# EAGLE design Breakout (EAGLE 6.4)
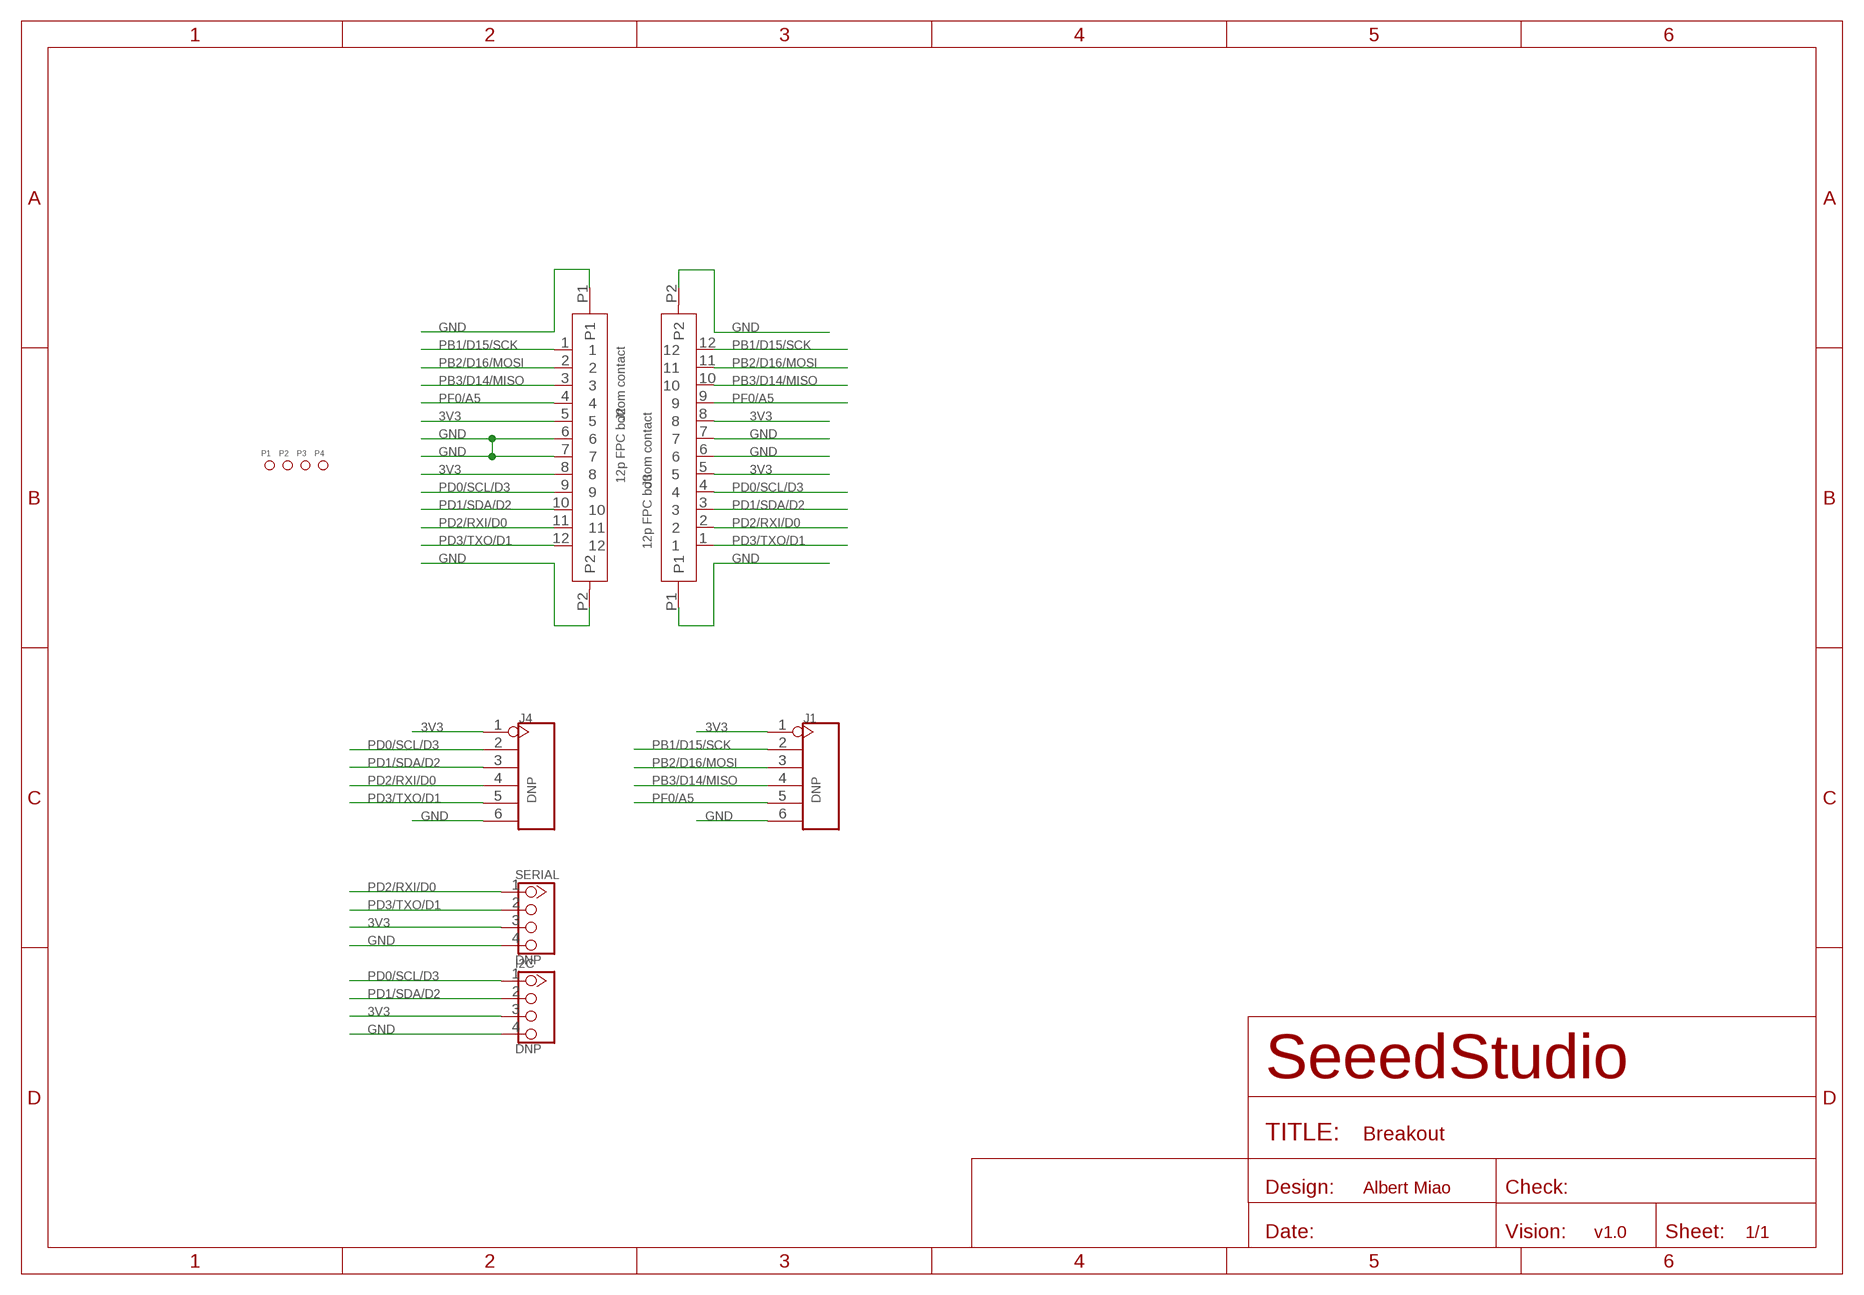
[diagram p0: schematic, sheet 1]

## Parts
I2C  DNP  TWIG-2.0-LEADED  [4P-LEADED-2.0]
J1  DNP  HEADER-6P-65/35MIL  [6P-2.54-65/35MIL]
J2  12p FPC bottom contact  FPC052002-12LT  [12P-0.5]
J3  12p FPC bottom contact  FPC052002-12LT  [12P-0.5]
J4  DNP  HEADER-6P-65/35MIL  [6P-2.54-65/35MIL]
P1  PAD-MARK  [ROUND-MARK-1.0]
P2  PAD-MARK  [ROUND-MARK-1.0]
P3  PAD-MARK  [ROUND-MARK-1.0]
P4  PAD-MARK  [ROUND-MARK-1.0]
SERIAL  DNP  TWIG-2.0-LEADED  [4P-LEADED-2.0]

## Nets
3V3: I2C.3 J1.1 J2.5 J2.8 J3.5 J3.8 J4.1 SERIAL.3
GND: I2C.4 J1.6 J2.6 J2.7 J2.P1 J2.P2 J3.6 J3.7 J3.P1 J3.P2 J4.6 SERIAL.4
PB1/D15/SCK: J1.2 J2.1 J3.12
PB2/D16/MOSI: J1.3 J2.2 J3.11
PB3/D14/MISO: J1.4 J2.3 J3.10
PD0/SCL/D3: I2C.1 J2.9 J3.4 J4.2
PD1/SDA/D2: I2C.2 J2.10 J3.3 J4.3
PD2/RXI/D0: J2.11 J3.2 J4.4 SERIAL.1
PD3/TXO/D1: J2.12 J3.1 J4.5 SERIAL.2
PF0/A5: J1.5 J2.4 J3.9

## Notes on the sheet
- Albert Miao
- v1.0

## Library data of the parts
I2C SERIAL = Connector:TWIG-2.0-LEADED
J1 J4 = Connector:HEADER-6P
J2 J3 = template:FPC052002-12LT
P1-P4 = Discrete:PAD-MARK; PARTNO: DNP

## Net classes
0 default: width 0.152 mm, drill 0.305 mm, clearance 0.152 mm
1 GND: width 0.152 mm, drill 0.305 mm, clearance 0.152 mm to class 0, clearance 0.152 mm
3 usbvcc: width 0.203 mm, drill 0.305 mm, clearance 0.203 mm

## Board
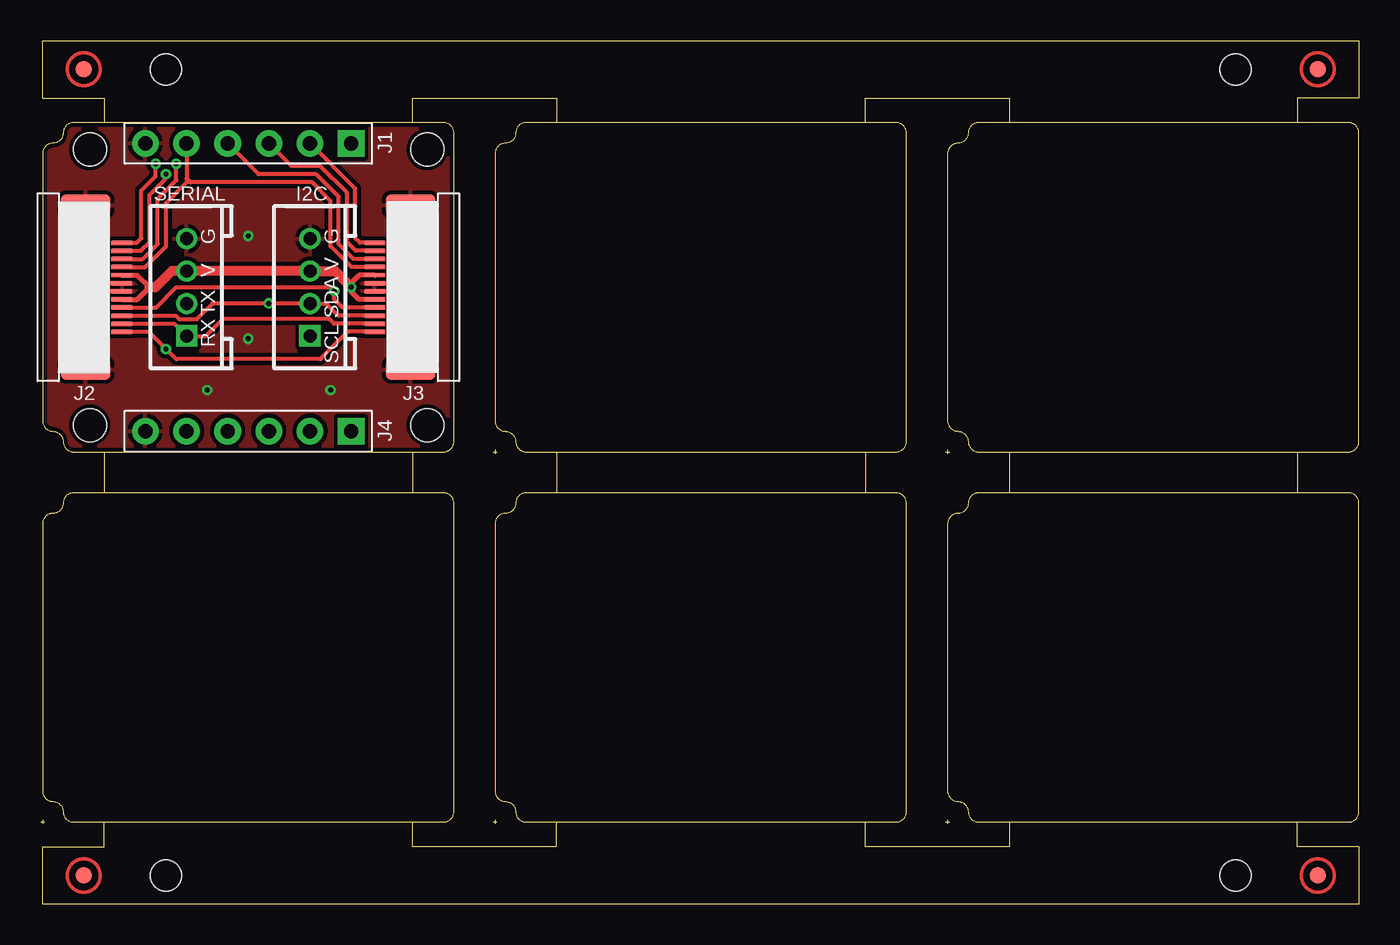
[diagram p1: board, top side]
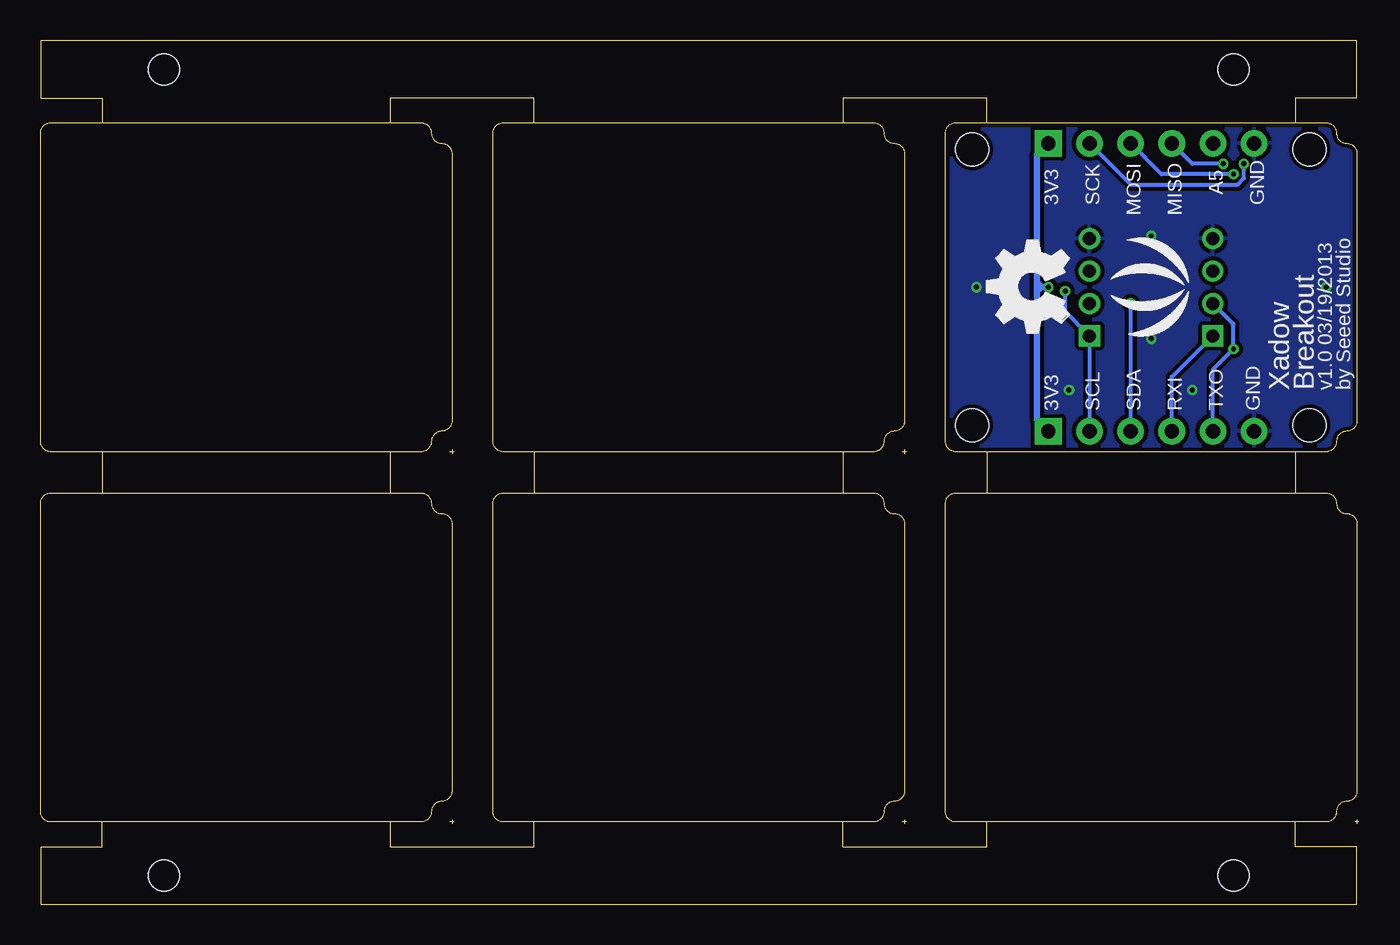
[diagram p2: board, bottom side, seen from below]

Size 81.41 x 53.34 mm. Coordinates in mm from the lower left corner, seen from the top.
Outline: 134 segments
Copper layers (1*16): Top 0.035mm / dielectric 1.5mm / Bottom 0.035mm
Design rules "SeeedStudio_rule_no_angle_090911": minimum track width 6mil, minimum drill 12mil, track to track 6mil, track to pad 6mil, pad to pad 6mil, via to via 6mil, smd to smd 0mil, copper to edge 10mil, drill to drill 10mil, minimum pad ring 10mil, minimum via ring 6mil, stop-mask expansion 2mil, vias tented up to drill 25mil, thermal gap 10mil
Holes 2.03 mm at 3.05,29.59 3.05,46.61 23.88,46.61 23.88,29.59
Holes 1.91 mm at 73.79,51.56 7.75,51.56 7.75,1.78 73.79,1.78
tRestrict: area 21,37.8 to 21.6,38.4; area 4.2,37.8 to 4.7,38.4

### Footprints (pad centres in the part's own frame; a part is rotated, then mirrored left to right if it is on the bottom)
4P-LEADED-2.0 = drill 0.8 pad 1.27 square: 1 -3,0 | drill 0.8 pad 1.27: 2 -1,0; 3 1,0; 4 3,0
6P-2.54-65/35MIL = drill 0.889 pad 1.651 square: 1 0,6.35 | drill 0.889 pad 1.651: 2 0,3.81; 3 0,1.27; 4 0,-1.27; 5 0,-3.81; 6 0,-6.35
12P-0.5 = smd 0.3 x 1.3: 1 -2.75,2.35; 2 -2.25,2.35; 3 -1.75,2.35; 4 -1.25,2.35; 5 -0.75,2.35; 6 -0.25,2.35; 7 0.25,2.35; 8 0.75,2.35; 9 1.25,2.35; 10 1.75,2.35; 11 2.25,2.35; 12 2.75,2.35 | smd 1.27 x 3.048: P1 -5.08,0.127; P2 5.08,0.127
ROUND-MARK-1.0 = smd 1.016 x 1.016: P$1 0,0

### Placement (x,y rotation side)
I2C  16.64,38.1 90 top
J1  12.83,46.99 270 top
J2  2.67,38.1 270 top
J3  22.99,38.1 90 top
J4  12.83,29.21 270 top
P1  2.67,51.56 0 top
P2  78.87,51.56 0 top
P3  2.67,1.78 0 top
P4  78.87,1.78 0 top
SERIAL  9.02,38.1 90 top
U$2  [LOGO_SILK]  12.19,38.1 90 bottom
U$3  [OSHW_FILLX200_NOTEXT]  17.91,35.31 90 bottom

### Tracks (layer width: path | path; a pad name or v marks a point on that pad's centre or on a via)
3V3  (via drill 0.3 pad 0.64)
  Top 0.305: J2.5 5.98,38.85 6.73,38.1 5.98,37.35 J2.8 | J3.8 19.67,38.85 19.18,38.35 v19.18,38.1 19.18,37.85 19.67,37.35 J3.5
  Top 0.61: 6.73,38.1 7.11,38.1 8.11,39.1 SERIAL.3 I2C.3 18.18,39.1 v19.18,38.1
  Bottom 0.406: J4.1 19.88,29.91 19.88,37.85 | 19.88,37.85 19.88,38.12 | 19.88,38.12 19.88,46.29 J1.1 | 19.88,38.12 19.6,38.12 | v19.18,38.1 19.2,38.12 19.58,38.12 | 19.58,38.12 19.81,38.35 | 19.58,38.12 19.6,38.12 | 19.6,38.12 19.88,37.85
GND  (via drill 0.3 pad 0.64)
  Top 0.254: J2.7 3.31,37.85 3.3,37.85 | J3.6 22.35,37.85 | J3.7 23.37,38.35 v23.62,38.1 | J2.6 2.28,38.35 v2.03,38.1
  other vias: 12.83,34.93 12.83,41.27 10.29,31.75 17.91,31.75
  pour Top (isolate 0.254): 0.13,27.94 25.53,27.94 25.53,48.26 0.13,48.26
  pour Bottom (isolate 0.254): 0.13,27.94 25.53,27.94 25.53,48.26 0.13,48.26
PB1/D15/SCK  (via drill 0.3 pad 0.64)
  Top 0.254: J3.12 19.73,40.85 19.43,41.15 19.43,44.2 J1.2 | J2.1 5.92,40.85 6.22,41.15 6.22,44.07 7.11,44.96 v7.11,45.72
  Bottom 0.254: J1.2 14.1,44.45 7.49,44.45 7.11,44.83 v7.11,45.72
PB2/D16/MOSI  (via drill 0.3 pad 0.64)
  Top 0.254: J3.11 19.47,40.35 18.92,40.89 18.92,43.94 17.27,45.59 15.49,45.59 J1.3 | J2.2 6.19,40.35 6.73,40.89 6.73,43.81 7.75,44.83 v7.75,45.09
  Bottom 0.254: v7.75,45.09 12.19,45.09 J1.3
PB3/D14/MISO  (via drill 0.3 pad 0.64)
  Top 0.254: J3.10 19.33,39.85 18.41,40.77 18.41,43.69 17.02,45.09 13.46,45.09 J1.4 | J2.3 6.32,39.85 7.24,40.77 7.24,43.56 8.38,44.7 v8.38,45.72
  Bottom 0.254: v8.38,45.72 10.29,45.72 J1.4
PD0/SCL/D3  (via drill 0.3 pad 0.64)
  Top 0.254: J2.9 7.13,36.85 8.38,38.1 17.91,38.1 v18.14,37.87 18.14,37.34 18.27,37.21 18.29,37.21 18.65,36.85 J3.4
  Bottom 0.254: I2C.1 J4.2 | I2C.1 | I2C.1 18.14,36.6 v18.14,37.87
PD1/SDA/D2  (via drill 0.3 pad 0.64)
  Top 0.254: J2.10 8.35,36.35 8.57,36.13 9.65,36.13 10.62,37.1 v14.1,37.1 I2C.2 17.64,37.1 18.39,36.35 J3.3
  Bottom 0.254: J4.3 v14.1,37.1
PD2/RXI/D0
  Top 0.254: J2.11 8.27,35.85 SERIAL.1 10.21,35.1 11.24,36.13 17.84,36.13 18.12,35.85 J3.2
  Bottom 0.254: J4.4 11.56,32.56 SERIAL.1
PD3/TXO/D1  (via drill 0.3 pad 0.64)
  Top 0.254: J2.12 6.69,35.35 v7.75,34.29 8.38,33.66 17.27,33.66 18.97,35.35 J3.1
  Bottom 0.254: SERIAL.2 7.75,35.83 v7.75,34.29 9.02,33.02 J4.5
PF0/A5
  Top 0.254: J3.9 19.2,39.35 17.91,40.64 17.91,43.43 16.76,44.58 9.27,44.58 | 9.27,44.58 9.02,44.58 | J2.4 6.46,39.35 7.75,40.64 7.75,43.31 9.02,44.58 | J1.5 9.02,44.83 | 9.02,44.83 9.02,44.58 | 9.27,44.58 9.02,44.83

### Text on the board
tPlace: G | G | V | V | TX | SDA | RX | SCL
bPlace: A5 | GND | SCK | 3V3 | MISO | MOSI | by Seeed Studio | v1.0 03/19/2013 | Breakout | Xadow | GND | TXO | RXI | SDA | SCL | 3V3
dxf: Unit:mm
